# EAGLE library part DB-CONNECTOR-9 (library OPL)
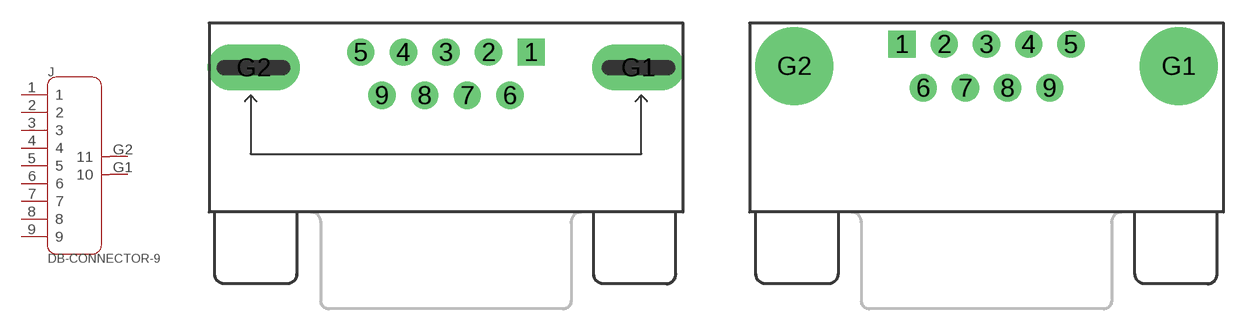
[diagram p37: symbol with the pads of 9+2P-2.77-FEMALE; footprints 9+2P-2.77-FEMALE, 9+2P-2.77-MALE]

Designator prefix J

## DB-CONNECTOR-9-320110019  [9+2P-2.77-FEMALE]
1  1
2  2
3  3
4  4
5  5
6  6
7  7
8  8
9  9
G1  10
G2  11

## DB-CONNECTOR-9-320110017  [9+2P-2.77-MALE]
Pads as for 9+2P-2.77-FEMALE

## Footprint 9+2P-2.77-FEMALE (pad centres in mm)
SUB-D
drill 1.143 pad 1.778 square: 1 5.54,0.9
drill 1.143 pad 1.778: 2 2.77,0.9; 3 0,0.9; 4 -2.77,0.9; 5 -5.54,0.9; 6 4.155,-1.91; 7 1.385,-1.91; 8 -1.385,-1.91; 9 -4.155,-1.91
drill 1 pad 3 long: G1 12.5,-0.1; G2 -12.5,-0.1

## Footprint 9+2P-2.77-MALE (pad centres in mm)
drill 1.143 pad 1.778 square: 1 -5.486,1.422
drill 1.143 pad 1.778: 2 -2.743,1.422; 3 0,1.422; 4 2.743,1.422; 5 5.486,1.422; 6 -4.115,-1.422; 7 -1.372,-1.422; 8 1.372,-1.422; 9 4.115,-1.422
drill 3.302 pad 5.08: G1 12.497,0; G2 -12.497,0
